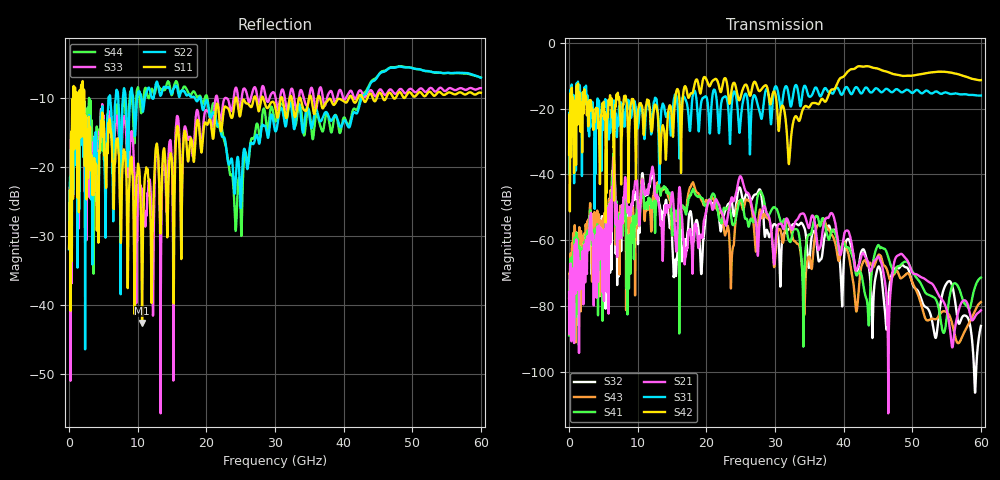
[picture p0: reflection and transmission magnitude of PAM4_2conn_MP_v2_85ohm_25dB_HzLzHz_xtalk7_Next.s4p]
! Info: Touchstone file created by Circ.  Input file=FAB50GbE_2conn_Midplane_Examax_Topo2_v2_85ohm_25dB_HzLzHz.circ
# Hz S RI R 50
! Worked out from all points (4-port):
!   6000 points, 10 MHz to 60 GHz, reference 50 ohm
!   strongest paths, dB at 10 MHz, 15.01 GHz, 30.01 GHz, 45.01 GHz, 60 GHz:
!     S42: -34.0, -24.0, -15.3, -7.9, -11.4
!     S31: -33.8, -23.5, -13.4, -14.2, -16.0
!     S21: -75.8, -45.5, -63.1, -65.0, -81.3
!     S41: -88.9, -58.1, -50.1, -61.5, -71.3
!     S43: -77.6, -53.0, -65.6, -64.7, -78.8
!     S32: -81.1, -59.3, -55.2, -68.2, -86.0
!   lowest |S11| = -42.5 dB at 10.64 GHz (marker M1), VSWR 1.02, Z = 49.6 - j0.636 ohm
!   |S11| at or under -10 dB: 2.217 GHz to 24.26 GHz (22.05 GHz wide, 167 % of centre); 28.28 GHz to 30.86 GHz (2.576 GHz wide, 8.71 % of centre); 36.56 GHz to 40.76 GHz (4.196 GHz wide, 10.9 % of centre)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
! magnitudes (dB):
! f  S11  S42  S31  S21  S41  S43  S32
! 10 MHz  -31.8  -34.0  -33.8  -75.8  -88.9  -77.6  -81.1
! 10.64 GHz  -42.5  -19.3  -20.0  -41.7  -41.9  -41.3  -39.9
! 15.43 GHz  -20.8  -17.7  -15.8  -57.7  -51.8  -52.0  -66.1
! 27.69 GHz  -11.9  -14.7  -20.4  -56.6  -45.7  -52.0  -44.6
! 32.07 GHz  -10.5  -36.3  -16.9  -55.1  -60.1  -55.6  -56.5
! 43.53 GHz  -9.9  -7.1  -14.0  -66.6  -81.0  -67.8  -66.9
! 60 GHz  -9.3  -11.4  -16.0  -81.3  -71.3  -78.8  -86.0
